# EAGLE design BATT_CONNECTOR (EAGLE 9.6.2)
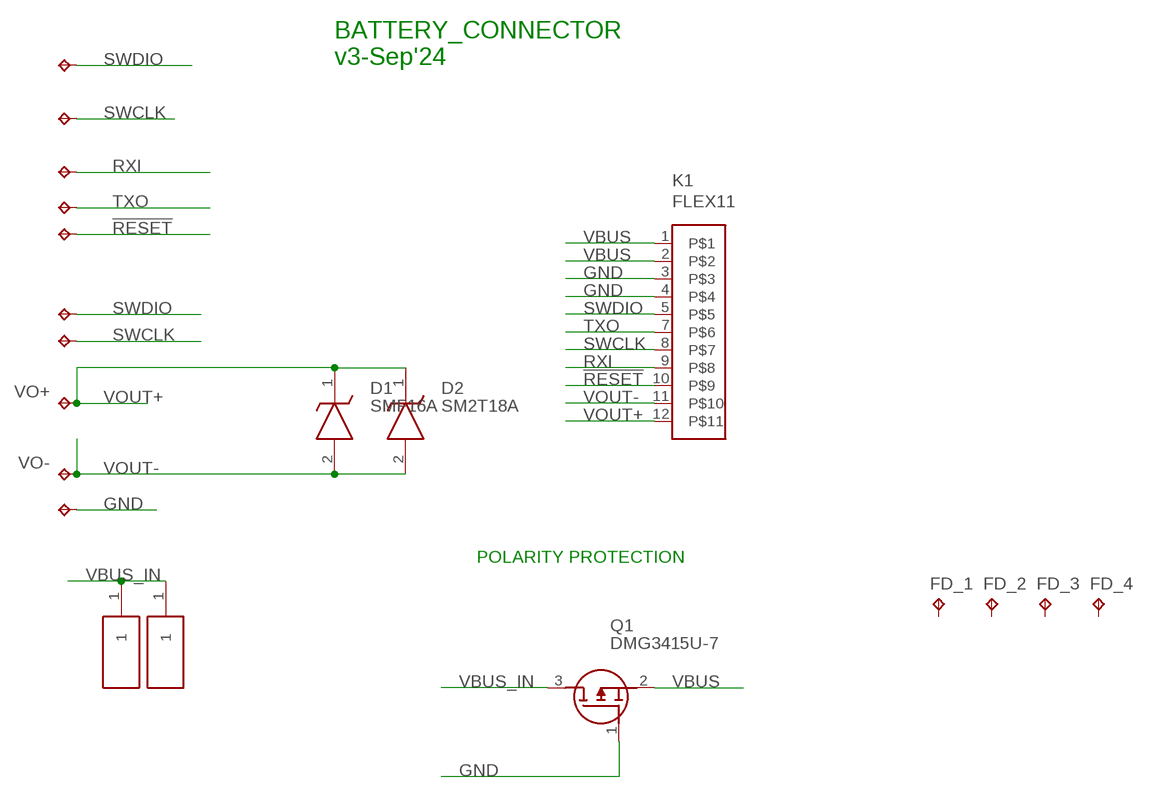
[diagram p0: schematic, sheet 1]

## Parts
!RESET  TPB2,54  [B2,54]
D1  SMF16A  [SODFL3618X110N]
D2  SM2T18A  [SM2T18A]
DAT  TPB2,54  [B2,54]
FD_1  FD_1  TPTP06SQ  [TP06SQ]
FD_2  FD_1  TPTP06SQ  [TP06SQ]
FD_3  FD_1  TPTP06SQ  [TP06SQ]
FD_4  FD_1  TPTP06SQ  [TP06SQ]
GND  TPB2,54  [B2,54]
H1  S1761-42R  [S176142R]
H2  S1761-42R  [S176142R]
ID  TPB2,54  [B2,54]
K1  FLEX11  [FLEX11]
Q1  DMG3415U-7  SSM3J338R,LF  [SSM3J332RLFT]
RXI  TPB2,54  [B2,54]
SWCLK  TPB2,54  [B2,54]
SWDIO  TPB2,54  [B2,54]
TXO  TPB2,54  [B2,54]
VO+  TPB2,54  [B2,54]
VO-  TPB2,54  [B2,54]

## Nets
!RESET: !RESET.TP K1.10
GND: GND.TP K1.3 K1.4 Q1.1(G)
RXI: K1.9 RXI.TP
SWCLK: ID.TP K1.8 SWCLK.TP
SWDIO: DAT.TP K1.5 SWDIO.TP
TXO: K1.7 TXO.TP
VBUS: K1.1 K1.2 Q1.2(S)
VBUS_IN: H1.1 H2.1 Q1.3(D)
VOUT+: D1.1(K) D2.1(K) K1.12 VO+.TP
VOUT-: D1.2(A) D2.2(A) K1.11 VO-.TP
Unconnected: FD_1.TP FD_2.TP FD_3.TP FD_4.TP

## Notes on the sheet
- BATTERY_CONNECTOR
  v3-Sep'24
- POLARITY PROTECTION

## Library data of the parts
!RESET DAT FD_1-FD_4 GND ID RXI SWCLK SWDIO TXO VO+ VO- = testpad:TP: Test pad
D1 = SMF16A:SMF16A: ESD Suppressors / TVS Diodes 200W 16V 5% Uni-directional; ARROW_PART_NUMBER: SMF16A; ARROW_PRICE-STOCK: https://www.arrow.com/en/products/smf16a/littelfuse; DESCRIPTION: ESD Suppressors / TVS Diodes 200W 16V 5% Uni-directional; HEIGHT: 1.1mm; MANUFACTURER_NAME: LITTELFUSE; MANUFACTURER_PART_NUMBER: SMF16A; MOUSER_PART_NUMBER: 576-SMF16A; MOUSER_PRICE-STOCK: https://www.mouser.co.uk/ProductDetail/Littelfuse/SMF16A?qs=IP%252BaFeBnnar8T%2Ffm%252BJ%2Flrw%3D%3D
D2 = SM2T18A:SM2T18A: 200 W TVS in STmite; DESCRIPTION: 200 W TVS in STmite; HEIGHT: 1.15mm; MANUFACTURER_NAME: STMicroelectronics; MANUFACTURER_PART_NUMBER: SM2T18A; MOUSER_PART_NUMBER: 511-SM2T18A; MOUSER_PRICE-STOCK: https://www.mouser.co.uk/ProductDetail/STMicroelectronics/SM2T18A?qs=9NrABl3fj%2FoQ9e7jVf8sKA%3D%3D
H1 H2 = S1761-42R:S1761-42R: EZ_Boardware SMT Spring Contact 3.5mm; DESCRIPTION: EZ_Boardware SMT Spring Contact 3.5mm; HEIGHT: 3.8mm; MANUFACTURER_NAME: Harwin; MANUFACTURER_PART_NUMBER: S1761-42R; MOUSER_PART_NUMBER: 855-S1761-42R; MOUSER_PRICE-STOCK: https://www.mouser.co.uk/ProductDetail/Harwin/S1761-42R?qs=ulE8k0yEMYZkmoaxRCFkSQ%3D%3D
K1 = Flex_3mm:FLEX11
Q1 = SSM3J338R_LF:SSM3J338R,LF: MOSFET Small-signal MOSFET Vdss= -12V, ID= -6A Source: Datasheet; ARROW_PART_NUMBER: SSM3J338R,LF; ARROW_PRICE-STOCK: https://www.arrow.com/en/products/ssm3j338rlf/toshiba?region=nac; DESCRIPTION: MOSFET Small-signal MOSFET Vdss= -12V, ID= -6A; HEIGHT: mm; MANUFACTURER_NAME: Toshiba; MANUFACTURER_PART_NUMBER: SSM3J338R,LF; MOUSER_PART_NUMBER: 757-SSM3J338RLF; MOUSER_PRICE-STOCK: https://www.mouser.co.uk/ProductDetail/Toshiba/SSM3J338RLF?qs=lhkzy8lC%252BSvURFM9ZjmJSw%3D%3D

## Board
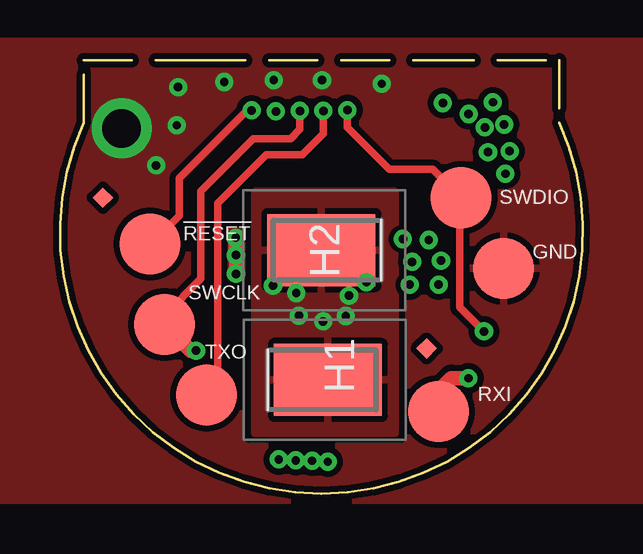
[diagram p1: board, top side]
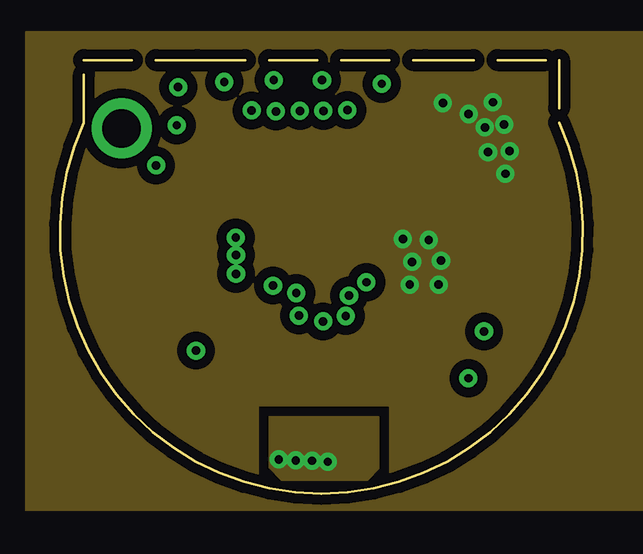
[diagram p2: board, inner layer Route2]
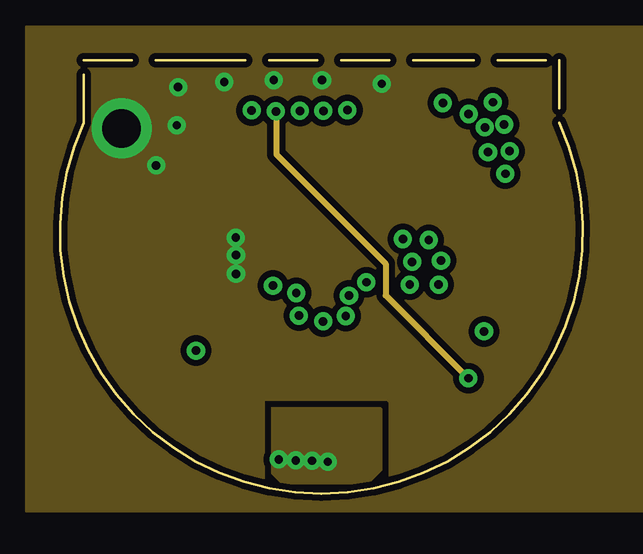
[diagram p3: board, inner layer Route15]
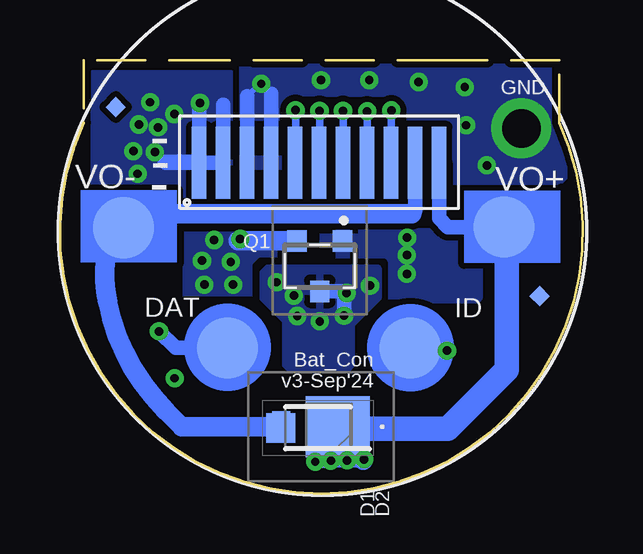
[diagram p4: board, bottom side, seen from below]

Size 21.79 x 18.07 mm. Coordinates in mm from the lower left corner, seen from the top.
Outline: 20.79,18.07 20.79,15.46 arc-229 0.99,15.46 0.99,18.07 5.73,18.07 5.71,18.06 15.21,18.06 15.23,18.07 20.79,18.07
Copper layers (1+2*15+16): Top 0.035mm / dielectric 1.5mm / Route2 0.035mm / dielectric 0.15mm / Route15 0.035mm / dielectric 0.2mm / Bottom 0.035mm
Design rules "default *": minimum track width 0.00038125mm, minimum drill 0.35mm, track to track 8mil, track to pad 8mil, pad to pad 8mil, via to via 8mil, smd to smd 5mil, copper to edge 8mil, drill to drill 8mil, minimum pad ring 10mil, minimum via ring 8mil, stop-mask expansion 2mil, vias tented up to drill 50mil, thermal gap 10mil
tRestrict: area 7.3,11.4 to 7.7,12.5; area 7.1,5.2 to 7.8,8.6
bRestrict: area 21,9.5 to 21.7,12.6; area 0.2,9.5 to 0.9,12.6

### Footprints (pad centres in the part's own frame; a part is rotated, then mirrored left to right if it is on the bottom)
B2,54 = smd 2.54 x 2.54: TP 0,0
SODFL3618X110N = smd 1.2 x 1.22: 1 -1.55,0; 2 1.55,0
SM2T18A = smd 2.67 x 2.54: 1 -0.698,0 | smd 0.762 x 1.27: 2 1.653,0
TP06SQ = smd 0.6 x 0.6: TP 0,0
S176142R = smd 3 x 4.5: 1 0,-2
FLEX11 = smd 0.6 x 3: 1 0.8,2.05; 2 1.8,2.05; 3 2.8,2.05; 4 3.8,2.05; 5 4.8,2.05; 7 5.8,2.05; 8 6.8,2.05; 9 7.8,2.05; 10 8.8,2.05; 11 9.8,2.05; 12 10.8,2.05
SSM3J332RLFT = smd 0.8 x 0.9: 1 -0.95,-1.05; 2 0.95,-1.05; 3 0,1.05

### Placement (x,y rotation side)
!RESET  3.74,10.41 0 top
D1  11.04,2.74 180 bottom
D2  10.91,2.79 180 bottom
DAT  14.81,6.07 0 bottom
FD_1  1.8,8.23 45 bottom
FD_2  19.46,16.11 45 bottom
FD_3  1.78,12.33 45 top
FD_4  15.27,6.05 45 top
GND  18.48,9.39 0 top
H1  13.16,4.74 270 top
H2  8.89,10.15 90 top
ID  7.19,6.07 0 bottom
K1  16.79,11.73 0 bottom
Q1  10.96,9.48 180 bottom
RXI  15.77,3.42 0 top
SWCLK  4.35,7.05 0 top
SWDIO  16.7,12.33 0 top
TXO  6.1,4.11 0 top
VO+  3.29,11.11 0 bottom
VO-  19.13,11.08 0 bottom

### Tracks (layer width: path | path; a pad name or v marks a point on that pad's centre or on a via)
!RESET  (via drill 0.35)
  Top 0.305: !RESET.TP 3.8,10.41 4.97,11.58 4.97,13.15 7.79,15.97 v7.98,15.97
  Bottom 0.203: K1.10
  Bottom 0.305: v7.98,15.97 K1.10
GND  (via drill 0.35, 1.6 pad 2.5)
  Top 0.61: v7.32,10.67 v7.32,9.95 v7.33,9.94 v7.33,9.16
  Bottom 0.203: 12.99,16.67 v13.4,17.08 13.47,17.08 13.99,16.56
  Bottom 0.61: 12.99,16.67 K1.4 | 13.99,16.56 K1.3
  other vias: 6.84,17.15 4,13.68 4.86,15.35 4.92,16.94 8.9,17.23 10.91,17.23 2.56,15.22
  pour Top (isolate 0.254, rank 2): -5.02,18.85 24.97,18.85 24.97,-0.28 -5.02,-0.28
  pour Route15 (isolate 0.254, rank 2): -1.42,19.46 -1.42,-0.74 25.06,-0.74 25.06,19.46
  pour Bottom (isolate 0.254, rank 2): 0.36,18.42 14.06,18.42 14.46,18.02 14.46,11.92 10.96,11.92 10.66,11.62 10.66,9.32 8.56,9.32 8.46,9.22 8.46,8.22 4.46,8.22 4.46,9.72 0.36,13.82
RXI  (via drill 0.35)
  Top 0.61: RXI.TP 15.77,4.28 16.3,4.81 v17.01,4.81
  Route15 0.203: v8.99,15.93 9.01,15.91
  Route15 0.254: v17.01,4.81 13.56,8.26 13.56,9.59 9.01,14.14 9.01,15.91
  Bottom 0.203: v8.99,15.93
  Bottom 0.305: K1.9 v8.99,15.93
SWCLK  (via drill 0.35)
  Top 0.254: SWCLK.TP 4.35,7.44
  Top 0.305: 4.35,7.44 5.86,8.95 5.86,12.6 8.05,14.79 9.6,14.79 9.99,15.18 v9.99,15.95 | 4.56,6.85 SWCLK.TP
  Top 0.61: v5.66,5.96 5.44,5.96 4.56,6.85
  Bottom 0.305: v9.99,15.95 K1.8
  Bottom 0.61: ID.TP 7.09,5.96 v5.66,5.96
SWDIO  (via drill 0.35)
  Top 0.305: v11.97,15.98 11.97,15.26 13.72,13.51 15.52,13.51 SWDIO.TP 16.66,12.29 16.66,7.76 v17.66,6.76
  Bottom 0.203: 11.97,13.8 K1.5
  Bottom 0.305: v11.97,15.98 11.97,13.8
  Bottom 0.61: DAT.TP 16.97,6.07 v17.66,6.76
TXO  (via drill 0.35)
  Top 0.305: TXO.TP 6.23,4.11 6.57,4.45 6.57,12.11 8.58,14.12 10.1,14.12 10.97,15 v10.97,15.95
  Bottom 0.203: 10.97,13.8 K1.7
  Bottom 0.305: v10.97,15.95 10.97,13.8
VBUS  (via drill 0.35)
  Bottom 0.61: v14.28,10.61 14.36,10.53 | 14.99,16.21 K1.2 17.38,13.78 17.42,13.82 16.03,13.82 K1.1 15.99,16.24 v15.95,16.28
  Bottom 0.813: Q1.2 14.36,10.53
  other vias: 18.03,16.31 17.02,15.82 17.83,14.23 18.73,14.27 18.5,15.38 14.67,9.66 15.36,10.57 15.87,9.71 18.55,13.33 17.7,15.26 15.77,8.71 14.57,8.71
  pour Route2 (isolate 0.406, rank 2): -1.44,19.22 -1.44,-0.68 25.07,-0.68 25.07,19.22
  pour Bottom (isolate 0.254): 14.63,17.62 14.63,12.13 20.46,12.13 20.46,17.62
  pour Bottom (isolate 0.305, rank 2): 12.77,8.24 16.63,8.24 16.63,11.22 12.77,11.22
VBUS_IN  (via drill 0.35)
  Bottom 0.61: Q1.3 10.06,8.43 9.95,8.32 v9.95,7.42
  other vias: 10.96,7.18 9.84,8.36 11.9,7.4 12.04,8.25 8.87,8.67 12.76,8.81
  pour Top: 8.1,12.59 13.96,12.59 13.96,2.51 8.1,2.51
  pour Bottom (isolate 0.254): 8.58,9.4 13.12,9.4 13.31,9.21 13.31,8.14 11.59,6.42 10.29,6.42 8.52,8.19 8.52,9.36 8.55,9.39
  pour Bottom: 9.56,7.32 9.56,5.32 9.76,5.12 12.16,5.12 12.26,5.12 12.46,5.32 12.46,7.32
VOUT+  (via drill 0.35)
  Bottom 0.61: v9.11,1.43 9.15,1.39 v9.82,1.39 10.48,1.39 v10.5,1.37 11.11,1.37 v11.15,1.33 | K1.12 5.99,11.48 5.62,11.11 VO+.TP
  Bottom 0.813: D1.1 10.17,2.74 D2.1 10.22,2.45 9.15,1.39
  Bottom 1.016: VO+.TP 3.16,10.98 3.16,5.17 5.63,2.71 9.46,2.71 D1.1
  pour Route2 (isolate 0.254): 8.71,1.1 9.22,0.59 12.81,0.59 13.27,1.05 13.27,3.19 8.71,3.19
  pour Route15 (isolate 0.254): 8.82,3.58 8.82,0.85 9.21,0.46 9.24,0.43 12.57,0.43 12.83,0.43 13.4,1 13.4,3.52 13.37,3.55 8.85,3.55
VOUT-
  Bottom 0.152: VO-.TP 19.17,11.12 19.56,11.12
  Bottom 0.61: K1.11 6.99,11.79 7.12,11.66
  Bottom 0.813: VO-.TP 18.55,11.66 7.12,11.66 | 19.56,11.12 arc-32 19.81,7.98 arc-34 17.38,3.46 16.71,2.79 D2.2 | D2.2 12.59,2.76 | D1.2 12.57,2.77 D2.2
(copper drawn outside any net)
  shapes: Bottom area x2, Bottom circle x2

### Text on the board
bPlace: Bat_Con / v3-Sep'24
bNames: GND | - | - | -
